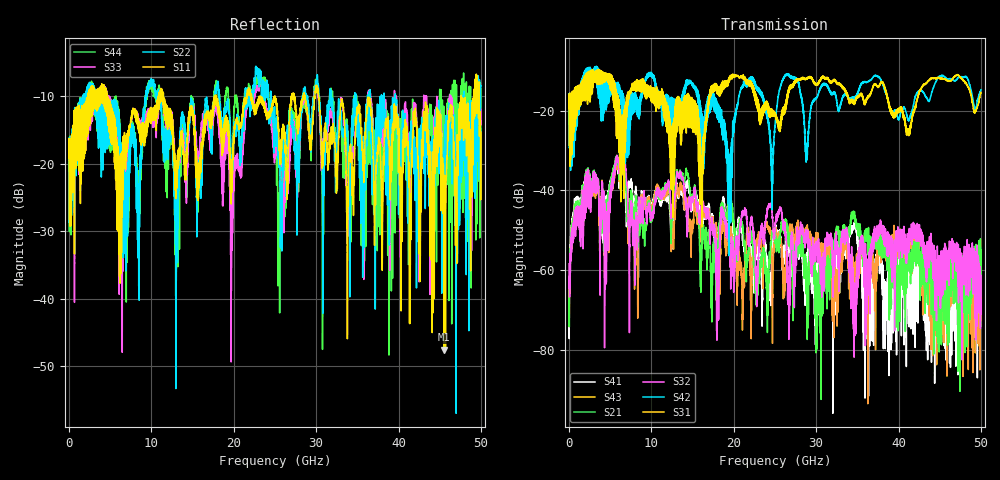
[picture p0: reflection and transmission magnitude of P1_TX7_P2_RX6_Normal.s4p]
!Keysight Technologies,N5225B,MY57041031,A.13.20.10
!Date: Friday, May 31, 2019 11:37:15
!Correction: S11(Full 4 Port(1,2,3,4))
!S12(Full 4 Port(1,2,3,4))
!S13(Full 4 Port(1,2,3,4))
!S14(Full 4 Port(1,2,3,4))
!S21(Full 4 Port(1,2,3,4))
!S22(Full 4 Port(1,2,3,4))
!S23(Full 4 Port(1,2,3,4))
!S24(Full 4 Port(1,2,3,4))
!S31(Full 4 Port(1,2,3,4))
!S32(Full 4 Port(1,2,3,4))
!S33(Full 4 Port(1,2,3,4))
!S34(Full 4 Port(1,2,3,4))
!S41(Full 4 Port(1,2,3,4))
!S42(Full 4 Port(1,2,3,4))
!S43(Full 4 Port(1,2,3,4))
!S44(Full 4 Port(1,2,3,4))
!S4P File: Measurements: <S11,S12,S13,S14>,
!<S21,S22,S23,S24>,
!<S31,S32,S33,S34>,
!<S41,S42,S43,S44>:
# Hz S  dB  R 50.0
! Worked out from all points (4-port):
!   5000 points, 10 MHz to 50 GHz, reference 50 ohm
!   strongest paths, dB at 10 MHz, 12.51 GHz, 25.01 GHz, 37.51 GHz, 50 GHz:
!     S31: -19.5, -39.3, -20.9, -14.0, -15.6
!     S42: -19.5, -16.9, -23.8, -11.5, -14.8
!     S32: -58.4, -44.6, -49.6, -49.4, -69.8
!     S21: -68.2, -45.6, -50.0, -50.7, -58.4
!     S43: -62.7, -48.9, -51.0, -55.5, -72.3
!     S41: -69.8, -51.5, -49.8, -55.2, -60.7
!   lowest |S11| = -47.5 dB at 45.52 GHz (marker M1), VSWR 1.01, Z = 49.7 + j0.305 ohm
!   |S11| at or under -10 dB: 4.613 GHz to 10.86 GHz (6.246 GHz wide, 80.7 % of centre); 11.46 GHz to 17.73 GHz (6.279 GHz wide, 43 % of centre); 30.28 GHz to 47.61 GHz (17.33 GHz wide, 44.5 % of centre)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
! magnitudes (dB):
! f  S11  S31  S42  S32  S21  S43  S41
! 10 MHz  -19.1  -19.5  -19.5  -58.4  -68.2  -62.7  -69.8
! 5.8 GHz  -29.0  -26.9  -15.4  -31.2  -31.2  -32.1  -32.1
! 19.46 GHz  -16.6  -12.3  -32.5  -53.8  -44.5  -49.3  -43.6
! 22.07 GHz  -10.5  -13.5  -11.6  -47.1  -50.2  -59.9  -54.1
! 24.67 GHz  -11.1  -20.3  -43.1  -46.9  -50.8  -67.2  -53.7
! 45.52 GHz  -47.5  -12.0  -11.4  -57.4  -58.5  -63.5  -62.3
! 50 GHz  -15.4  -15.6  -14.8  -69.8  -58.4  -72.3  -60.7
